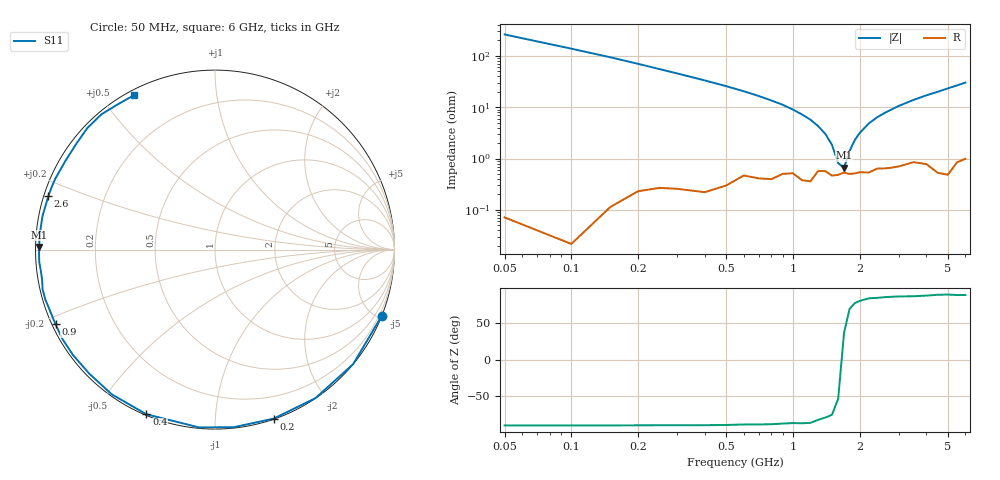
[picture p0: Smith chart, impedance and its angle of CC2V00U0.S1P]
! Infineon Technologies  Discrete & RF Semiconductors
! BBY57-02W
! Si Tuning Diode in SCD-80
! VR = 2 V
! S-Parameters:  June  2000
# GHz  S  MA  R  50
!  f  S11
! GHz  MAG  ANG
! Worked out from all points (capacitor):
!   34 points, 50 MHz to 6 GHz, reference 50 ohm
!   read as one part to ground: C = 11.4 pF near 50 MHz
!   lowest |Z| = 662 mohm at 1.7 GHz (marker M1)
!   series resonance near 1.663 GHz, so ESL is about 800 pH
!   S11 on the Smith chart (normalised r, x): 50 MHz: 0.00, -5.24; 200 MHz: 0.00, -1.40; 400 MHz: 0.00, -0.67; 900 MHz: 0.01, -0.22; 2.6 GHz: 0.01, +0.16; 6 GHz: 0.02, +0.60
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0.05  0.9999 -21.6
0.1  0.9999 -39.7
0.15  0.999 -55.9
0.2  0.9969 -70.9
0.25  0.9952 -84.1
0.3  0.9944 -95.2
0.4  0.9939 -112.6
0.5  0.9906 -125.5
0.6  0.9841 -135.4
0.7  0.9853 -143.3
0.8  0.9853 -149.7
0.9  0.981 -154.9
1  0.9802 -159.6
1.1  0.9853 -163.6
1.2  0.9859 -167.0
1.3  0.9775 -170.3
1.6  0.9809 -178.5
1.7  0.9789 179.1
2.2  0.979 169.0
2.4  0.9752 165.5
2.6  0.9752 162.3
3  0.9735 156.1
3.5  0.9689 149.0
4  0.9724 142.3
4.5  0.982 136.4
5  0.9842 130.0
5.5  0.974 123.9
6  0.9714 117.7
